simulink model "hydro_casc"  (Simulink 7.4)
settings: Solver=ode45  StartTime=0.0  StopTime=400  MaxStep=1  RelTol=1e-3
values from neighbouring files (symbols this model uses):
  k = 0.7    [ZRS1_Primer4_11.m]    (also in basic_control.m = 2; basic_control_1.m = 2; main_hydro.m = [100 1 1]; optimise.m = 5)
undefined symbols (not defined in the file or in its folder): Hydro_for_Matlab21, newDymolaGui
libraries: simulink_extras x1

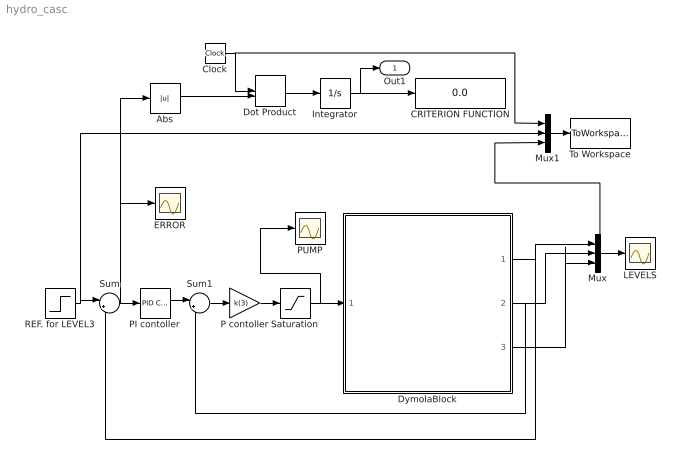
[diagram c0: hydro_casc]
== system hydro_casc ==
  Abs : Abs
  CRITERION FUNCTION : Display
  Clock : Clock
  Dot Product : DotProduct  OutDataType=sfix(16)  OutScaling=2^-10
  DymolaBlock : Subsystem  Tag=28-Jan-2005 21:14:21#9501
  ERROR : Scope
  Integrator : Integrator
  LEVELS : Scope
  Mux : Mux  Inputs=3
  Mux1 : Mux  Inputs=3
  P contoller : Gain  Gain=k(3)  ParameterDataType=sfix(16)  ParameterScaling=2^0  OutDataType=sfix(16)  OutScaling=2^0
  PI contoller : simulink_extras/Additional Linear/PID Controller (with Approximate Derivative)  SystemSampleTime=-1  P=k(1)  I=k(2)  D=0  N=0.1
  PUMP : Scope
  REF. for LEVEL3 : Step  Time=0  After=0.1  SampleTime=0
  Saturation : Saturate  UpperLimit=10  LowerLimit=0
  Sum : Sum  Inputs=|+-  OutDataType=sfix(16)  OutScaling=2^0
  Sum1 : Sum  Inputs=|+-  OutDataType=sfix(16)  OutScaling=2^0
  To Workspace : ToWorkspace  VariableName=levels  SampleTime=-1  SaveFormat=Array
  Out1 : Outport  OutDataType=sfix(16)  OutScaling=2^0
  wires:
  REF. for LEVEL3/1 -> Sum/1, Mux1/2
  Sum/1 -> PI contoller/1, ERROR/1, Abs/1
  Abs/1 -> Dot Product/2
  Clock/1 -> Dot Product/1, Mux1/1
  Dot Product/1 -> Integrator/1
  Mux1/1 -> To Workspace/1
  Integrator/1 -> CRITERION FUNCTION/1, Out1/1
  Mux/1 -> LEVELS/1, Mux1/3
  Sum1/1 -> P contoller/1
  PI contoller/1 -> Sum1/1
  Saturation/1 -> PUMP/1, DymolaBlock/1(InPort1)
  P contoller/1 -> Saturation/1
  DymolaBlock/1(OutPort1) -> Mux/1, Sum/2
  DymolaBlock/2(OutPort2) -> Mux/2, Sum1/2
  DymolaBlock/3(OutPort3) -> Mux/3

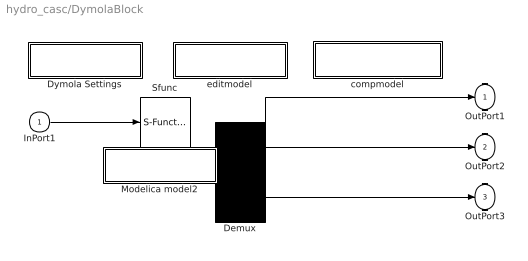
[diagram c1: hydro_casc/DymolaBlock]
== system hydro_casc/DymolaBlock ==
  InPort1 : Inport
  Demux : Demux  Outputs=[1;1;1]
  Dymola Settings : Subsystem  mask{ModelName=Hydro_for_Matlab21, MoFileName=C:/Users/bore/Documents/Dymola/Hydraulics/Hydro_for_Matlab21.mo, dSpace=, BusConnector=, ResultFile=, ResultFileOnline=, ResultDt=, Libs=:, bigobj=}
      mask prompts: ModelName "Name of Dymola model"; MoFileName "File Name (including .mo)"; ResultFile "Create Result"; ResultFileOnline "Load result"; ResultDt "Result min dt"; Libs "Used Libraries"; bigobj "Compiler flag /bigobj"
  Modelica model2 : Subsystem
  Sfunc : S-Function  Tag=950134qzx  FunctionName=hydro_for_matla_dy950134qzx  Parameters=[tank1_area;tank1_hr;tank1_h1;tank1_h3;tank1_hc1;tank1_hc2;tank1_hc3;tank1_beginninglevel;tank2_area;tank2_hr;tank2_h1;tank2_h3;tank2_hc1;tank2_hc2;tank2_hc3;tank2_beginninglevel;tank3_area;tank3_hr;tank3_h1;tank3_h3;tank3_hc1;tank3_hc2;tank3_hc3;tank3_beginninglevel;V12_sv;V12_kv;V23_sv;V23_kv;Valve4_sv;Valve4_kv;Valve5_sv;Valve5_kv;V3izh_sv;V3izh_kv;tank_area;tank_hr;tank_h1;tank_h3;tank_hc1;tan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  PortCounts=[1;1]  EnableBusSupport=off  mask{tank1_area=0.0154, tank1_hr=0.63, tank1_h1=0, tank1_h3=0, tank1_hc1=0, tank1_hc2=0, tank1_hc3=0, tank1_beginninglevel=0, tank2_area=0.0154, tank2_hr=0.63, tank2_h1=0, tank2_h3=0, tank2_hc1=0, tank2_hc2=0, tank2_hc3=0, tank2_beginninglevel=0, tank3_area=0.0154, tank3_hr=0.63, tank3_h1=0, tank3_h3=0, tank3_hc1=0, tank3_hc2=0, tank3_hc3=0, tank3_beginninglevel=0, V12_sv=1, V12_kv=0.0001, V23_sv=1, V23_kv=0.0001, Valve4_sv=0.1, Valve4_kv=0.0001, Valve5_sv=0, Valve5_kv=0.0001, V3izh_sv=1, V3izh_kv=0.0001, tank_area=1, tank_hr=0.25, tank_h1=0, tank_h3=0, tank_hc1=0, tank_hc2=0, tank_hc3=0, tank_beginninglevel=0.2, CPump1_hc=1.37, CPump1_k=1, flowelement1_area=2e-005, CValve1_kv=0.0001, Disturbance_height=0.2, Disturbance_offset=0, Disturbance_startTime=200, tank1_level=0, tank2_level=0, tank3_level=0, tank_level=0}
      mask prompts: tank1_area "tank1.area"; tank1_hr "tank1.hr"; tank1_h1 "tank1.h1"; tank1_h3 "tank1.h3"; tank1_hc1 "tank1.hc1"; tank1_hc2 "tank1.hc2"; tank1_hc3 "tank1.hc3"; tank1_beginninglevel "tank1.beginninglevel"; tank2_area "tank2.area"; tank2_hr "tank2.hr"; tank2_h1 "tank2.h1"; tank2_h3 "tank2.h3"; tank2_hc1 "tank2.hc1"; tank2_hc2 "tank2.hc2"; tank2_hc3 "tank2.hc3"; tank2_beginninglevel "tank2.beginninglevel"; tank3_area "tank3.area"; tank3_hr "tank3.hr"; tank3_h1 "tank3.h1"; tank3_h3 "tank3.h3"; tank3_hc1 "tank3.hc1"; tank3_hc2 "tank3.hc2"; tank3_hc3 "tank3.hc3"; tank3_beginninglevel "tank3.beginninglevel"; V12_sv "V12.sv"; V12_kv "V12.kv"; V23_sv "V23.sv"; V23_kv "V23.kv"; Valve4_sv "Valve4.sv"; Valve4_kv "Valve4.kv"; Valve5_sv "Valve5.sv"; Valve5_kv "Valve5.kv"; V3izh_sv "V3izh.sv"; V3izh_kv "V3izh.kv"; tank_area "tank.area"; tank_hr "tank.hr"; tank_h1 "tank.h1"; tank_h3 "tank.h3"; tank_hc1 "tank.hc1"; tank_hc2 "tank.hc2"; tank_hc3 "tank.hc3"; tank_beginninglevel "tank.beginninglevel"; CPump1_hc "CPump1.hc"; CPump1_k "CPump1.k"; flowelement1_area "flowelement1.area"; CValve1_kv "CValve1.kv"; Disturbance_height "Disturbance.height"; Disturbance_offset "Disturbance.offset"; Disturbance_startTime "Disturbance.startTime"; tank1_level "tank1.level"; tank2_level "tank2.level"; tank3_level "tank3.level"; tank_level "tank.level"
  compmodel : Subsystem  InitFcn=newDymolaGui('hydro_casc/DymolaBlock','Verify');
  editmodel : Subsystem
  OutPort1 : Outport
  OutPort2 : Outport  Port=2
  OutPort3 : Outport  Port=3
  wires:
  Sfunc/1 -> Demux/1
  Demux/1 -> OutPort1/1
  Demux/2 -> OutPort2/1
  Demux/3 -> OutPort3/1
  InPort1/1 -> Sfunc/1

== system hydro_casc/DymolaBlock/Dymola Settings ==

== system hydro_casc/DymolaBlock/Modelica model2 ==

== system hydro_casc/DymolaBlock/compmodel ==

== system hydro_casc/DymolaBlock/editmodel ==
